// TwinCAT 3 PLC project TCPCP_Client_SampleCode
// ProgramVersion: 3.1.0.9
// libraries:
//   Tc2_Standard, * (Beckhoff Automation GmbH)
//   Tc2_System, * (Beckhoff Automation GmbH)
//   Tc2_TcpIp, * (Beckhoff Automation GmbH)
//   Tc3_Interfaces, * (Beckhoff Automation GmbH)
//   Tc3_Module, * (Beckhoff Automation GmbH)
// project tree:
//   / PlcTask.TcTTO
//   POUs/ MAIN.TcPOU

CONFIGURATION TCPCP_Client_SampleCode
    RESOURCE PLC ON TwinCAT3
        TASK PlcTask(INTERVAL := T#10ms, PRIORITY := 20);
        PROGRAM MAIN WITH PlcTask : MAIN;
    END_RESOURCE
END_CONFIGURATION

// ---- POUs/MAIN.TcPOU
PROGRAM MAIN
VAR
	fbSocketConnect   	: FB_SocketConnect;(*TCP/IP建立连接的功能块*)
	fbSocketSend      	: FB_SocketSend;(*TCP/IP的发送功能块*)
	fbSocketReceive   	: FB_SocketReceive;(*TCP/IP的写入的功能块*)
	fbSocketClose     	: FB_SocketClose;(*TCP/IP的关闭建立连接的功能块*)
    bExecute          	: BOOL;(*TCP/IP建立连接的执行位*)
    hSocket           	: T_HSOCKET;(*TCP/IP的句柄*)
	arrSendData			: ARRAY[1..4] OF WORD := [16#1111, 16#2222, 16#3333, 16#4444];(*TCP/IP发送数组*)
	bSend				: BOOL;(*TCP/IP发送的执行位*)
	bRecieve          	: BOOL;(*TCP/IP接收的执行位*)
	arrRecieveData    	: ARRAY[1..4] OF WORD;(*TCP/IP接收数组*)
	bClose            	: BOOL;(*TCP/IP关闭连接的执行位*)
END_VAR

/////////////////////////////////////////////////////////
//注意：/////////////////////////////////////////////////
//该例程序仅供初学者入门学习使用/////////////////////////
//差错在所难免，无法保证绝对正确并完全满足您的使用需求///
//欢迎您提出改进建议。联系邮箱：Support@Beckhoff.com.cn//
/////////////////////////////////////////////////////////

fbSocketConnect(
	sSrvNetId:= , 
	sRemoteHost:='169.254.0.1', //TCP/IP Server的IP地址169.254.0.1
	nRemotePort:=6000 , 		//TCP/IP Server的I端口号6000
	bExecute:= bExecute, 		//TCP/IP连接的执行位*)
	tTimeout:=T#1S , 
	bBusy=> , 
	bError=> , 
	nErrId=> , 
	hSocket=>hSocket );			//通过SocketConnect获取句柄，供后续FB使用
	
fbSocketSend(
	sSrvNetId:= , 
	hSocket:=hSocket , 			//TCP/IP的句柄
	cbLen:=SIZEOF(arrSendData) ,//TCP/IP发送数据的长度
	pSrc:=ADR (arrSendData), 	//TCP/IP发送数据的指针起始地址
	bExecute:=bSend, 			//TCP/IP发送的执行位
	tTimeout:= T#1S, 
	bBusy=> , 
	bError=> , 
	nErrId=> );
	
fbSocketReceive(
	sSrvNetId:= , 
	hSocket:=hSocket , 				//TCP/IP的句柄
	cbLen:=SIZEOF(arrRecieveData) , //TCP/IP接收数据的长度
	pDest:=ADR (arrRecieveData) , 	//TCP/IP接收数据的指针起始地址
	bExecute:=bRecieve, 			//TCP/IP接收的执行位
	tTimeout:= T#1S , 
	bBusy=> , 
	bError=> , 
	nErrId=> , 
	nRecBytes=> );
	
fbSocketClose(
	sSrvNetId:= , 
	hSocket:=hSocket , 			//TCP/IP的句柄
	bExecute:=bClose , 			//TCP/IP关闭连接执行位
	tTimeout:=T#1S , 
	bBusy=> , 
	bError=> , 
	nErrId=> );

END_PROGRAM
